FUNCTION_BLOCK FB_DeleteProductById
VAR_IN_OUT
	fbClient:FB_IotHttpClient;
END_VAR
VAR_OUTPUT
	bBusy:BOOL;
	bError:BOOL;
	
END_VAR
VAR
	fbRequest			: FB_IotHttpRequest;
	fbJsonSend			: FB_JsonDomParser;
	jsonDoc				: SJsonValue;
	nState				: UDINT;
	DeleteRisingEdge			: R_TRIG;
	fbGetProductByBarCode:FB_GetProductByBarCode;
	domParse:FB_JsonDomParser;
	sUri:STRING;
END_VAR

//HMI
VAR
	bSend:BOOL;
	nStatusCode:UINT;
	deleteProductId:DINT;
END_VAR

DeleteRisingEdge(CLK:=bSend , Q=> );
CASE nState OF
	0:
		
		IF DeleteRisingEdge.Q AND deleteProductId<>0 THEN
			nStatusCode:=0;
			nState:=10;
			bBusy:=TRUE;
			bError:=FALSE;
		END_IF
	
		
	10:
		sUri:=CONCAT('/Product/',DINT_TO_STRING(deleteProductId));
		IF fbRequest.SendRequest(sUri:=sUri,fbClient:=fbClient,eRequestType:=ETcIotHttpRequestType.HTTP_DELETE,0,0,0) THEN
			nState:=20;
		END_IF
	20:
		IF NOT fbRequest.bBusy THEN
			nStatusCode:=fbRequest.nStatusCode;
			IF nStatusCode=200 THEN
				deleteProductId:=0;
			END_IF
			nState:=100;
		END_IF
		
	100:
		bBusy:=FALSE;
		nState:=0;
END_CASE

END_FUNCTION_BLOCK
